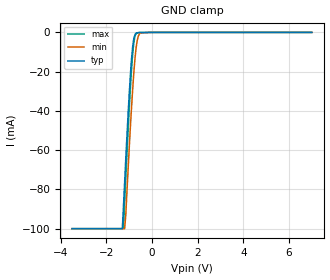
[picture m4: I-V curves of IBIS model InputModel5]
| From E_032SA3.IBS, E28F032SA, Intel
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|*************************Input Model 5****************************
[Model]   InputModel5
Model_type   Input
|   For CE#1
Vinl = 0.8V
Vinh = 2.0V
| Variable   typ   min   max
C_comp   5.61p   NA   7.6p
[Voltage Range]   3.3V   3.0V   3.6V
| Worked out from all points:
|   GND clamp passes 1 mA (typ) near -0.74 V on its own axis
[GND_clamp]
|Voltage I(typ)   I(min)   I(max)
-3.5V     -100mA     -100mA     -100mA
-1.3V     -100mA     -100mA     -100mA
-1.25V    -88.47mA   -100mA     -99.13mA
-1.2V     -76.42mA   -100mA     -86.6mA
-1.15V    -64.56mA   -93mA      -74.23mA
-1V       -31.64mA   -59.24mA   -39.42mA
-900mV    -13.8mA    -38.62mA   -19.43mA
-800mV    -3.214mA   -20.98mA   -5.547mA
-700mV    -419.8uA   -8.087mA   -691.1uA
-600mV    -110uA     -1.896mA   -166.7uA
-500mV    -24.25uA   -281.9uA   -46.34uA
7V        0A         0A         0A
[POWER_clamp]
| Input buffer circuits of this product do not intrinsically
| require a [POWER_clamp] definition.  This zero current
| [POWER_clamp] is provided for compatibility with some ibis
| parsers.
|   Voltage  I(typ)   I(min)   I(max)
-5V       0A         0A         0A
-4.75V    0A         0A         0A
9.75V     0A         0A         0A
10V       0A         0A         0A
